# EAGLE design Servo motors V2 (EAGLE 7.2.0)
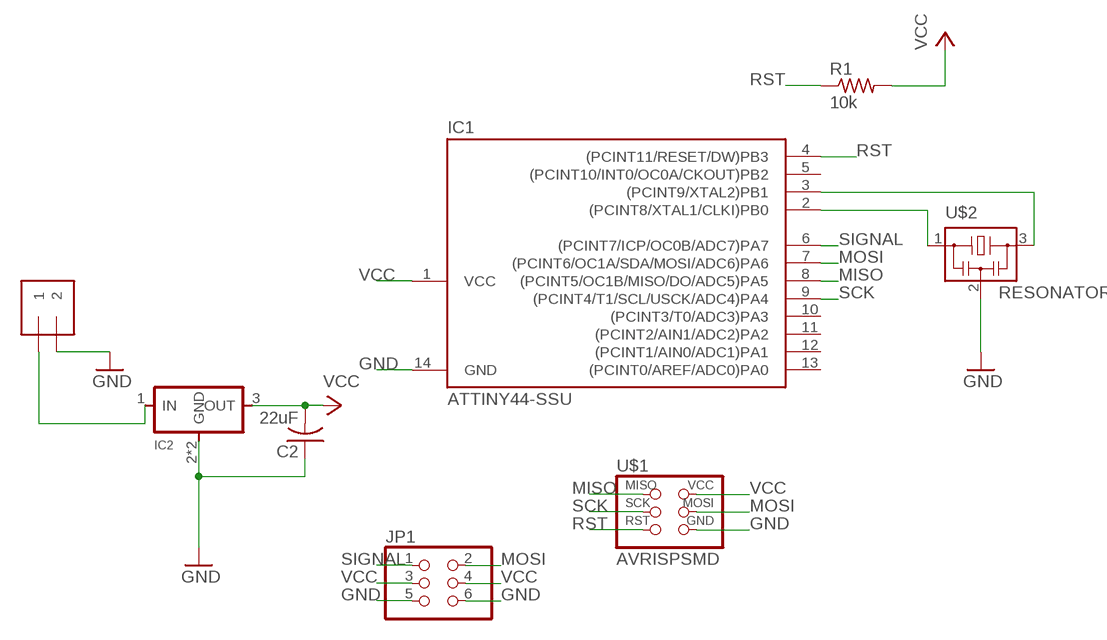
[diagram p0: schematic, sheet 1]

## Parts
C2  22uF  C-USC1206  [C1206]
IC1  ATTINY44-SSU  [SOIC14]
IC2  REGULATORSOT223  [SOT223]
J1  1X2-3.5MM  [3.5MMTERM]
JP1  PINHD-2X3-SMD  [2X03SMD]
R1  10k  RESISTOR1206  [1206]
U$1  AVRISPSMD  [2X03SMD]
U$2  RESONATOR  [EFOBM]

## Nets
GND: C2.1 IC1.14(GND) IC2.2(GND) IC2.4(GND) J1.2 JP1.5 JP1.6 U$1.6(GND) U$2.2
MISO: IC1.8((PCINT5/OC1B/MISO/DO/ADC5)PA5) U$1.1(MISO)
MOSI: IC1.7((PCINT6/OC1A/SDA/MOSI/ADC6)PA6) JP1.2 U$1.4(MOSI)
N$1: IC1.3((PCINT9/XTAL2)PB1) U$2.3
N$2: IC1.2((PCINT8/XTAL1/CLKI)PB0) U$2.1
N$3: IC2.1(IN) J1.1
RST: IC1.4((PCINT11/RESET/DW)PB3) R1.1 U$1.5(RST)
SCK: IC1.9((PCINT4/T1/SCL/USCK/ADC4)PA4) U$1.3(SCK)
SIGNAL: IC1.6((PCINT7/ICP/OC0B/ADC7)PA7) JP1.1
VCC: C2.2 IC1.1(VCC) IC2.3(OUT) JP1.3 JP1.4 R1.2 U$1.2(VCC)
Unconnected: IC1.5((PCINT10/INT0/OC0A/CKOUT)PB2) IC1.10((PCINT3/T0/ADC3)PA3) IC1.11((PCINT2/AIN1/ADC2)PA2) IC1.12((PCINT1/AIN0/ADC1)PA1) IC1.13((PCINT0/AREF/ADC0)PA0)

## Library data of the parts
C2 = 01_adafruit:C-US: CAPACITOR, American symbol
IC1 = 01_FAB_Hello:ATTINY44
IC2 = 01_fab:REGULATOR
J1 = 01_adafruit:1X2: 3.5mm Terminal block
JP1 = 01_FAB_Hello:PINHD-2X3-SMD: PIN HEADER
R1 = 01_FAB_Hello:RESISTOR
U$1 = 01_FAB_Hello:AVRISP
U$2 = 01_fab:RESONATOR

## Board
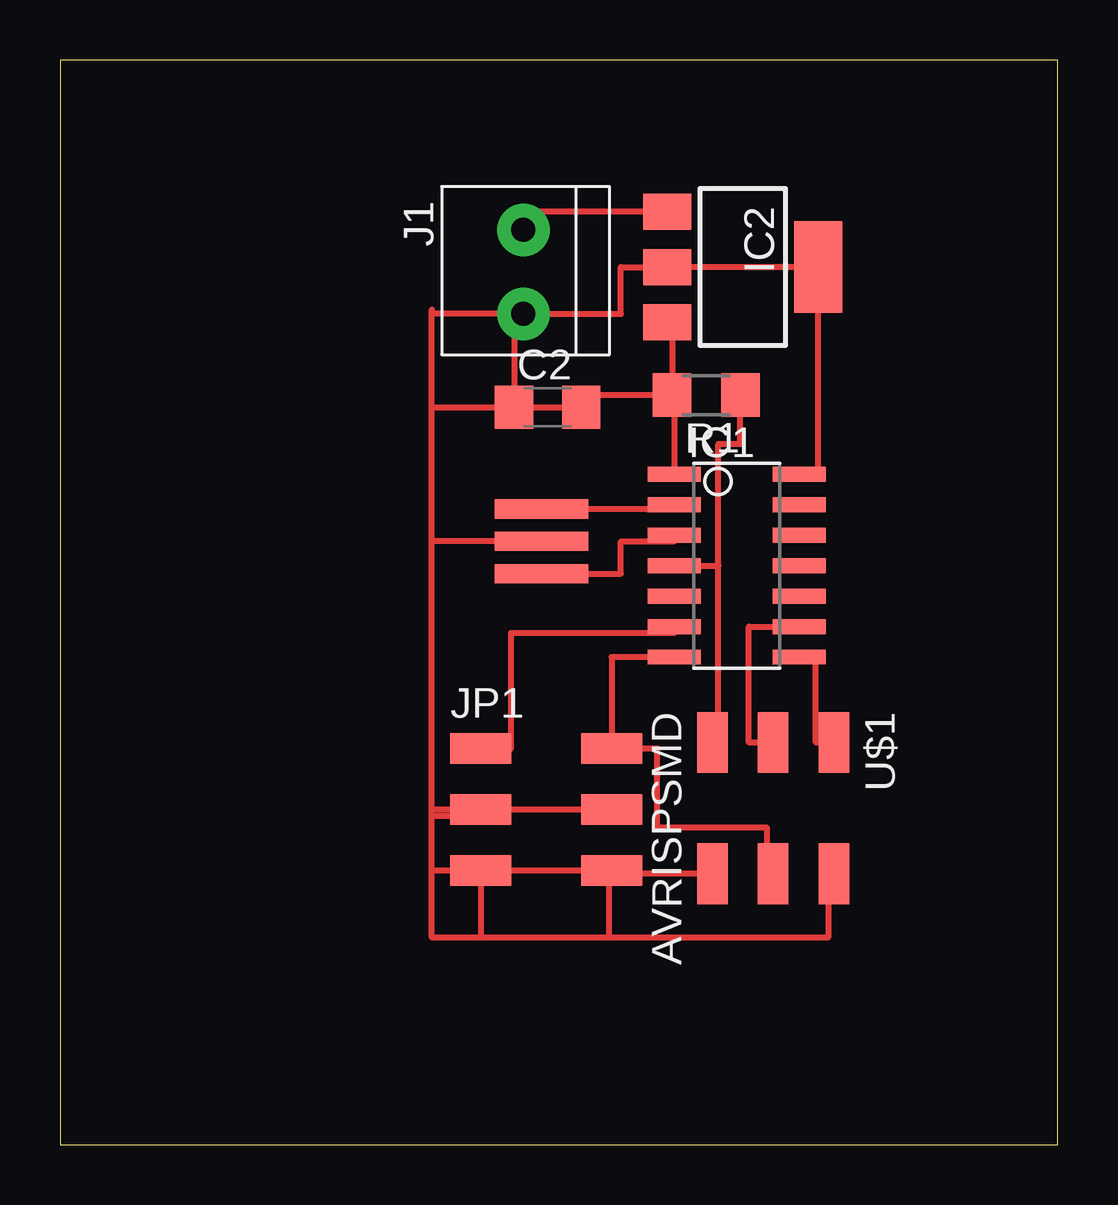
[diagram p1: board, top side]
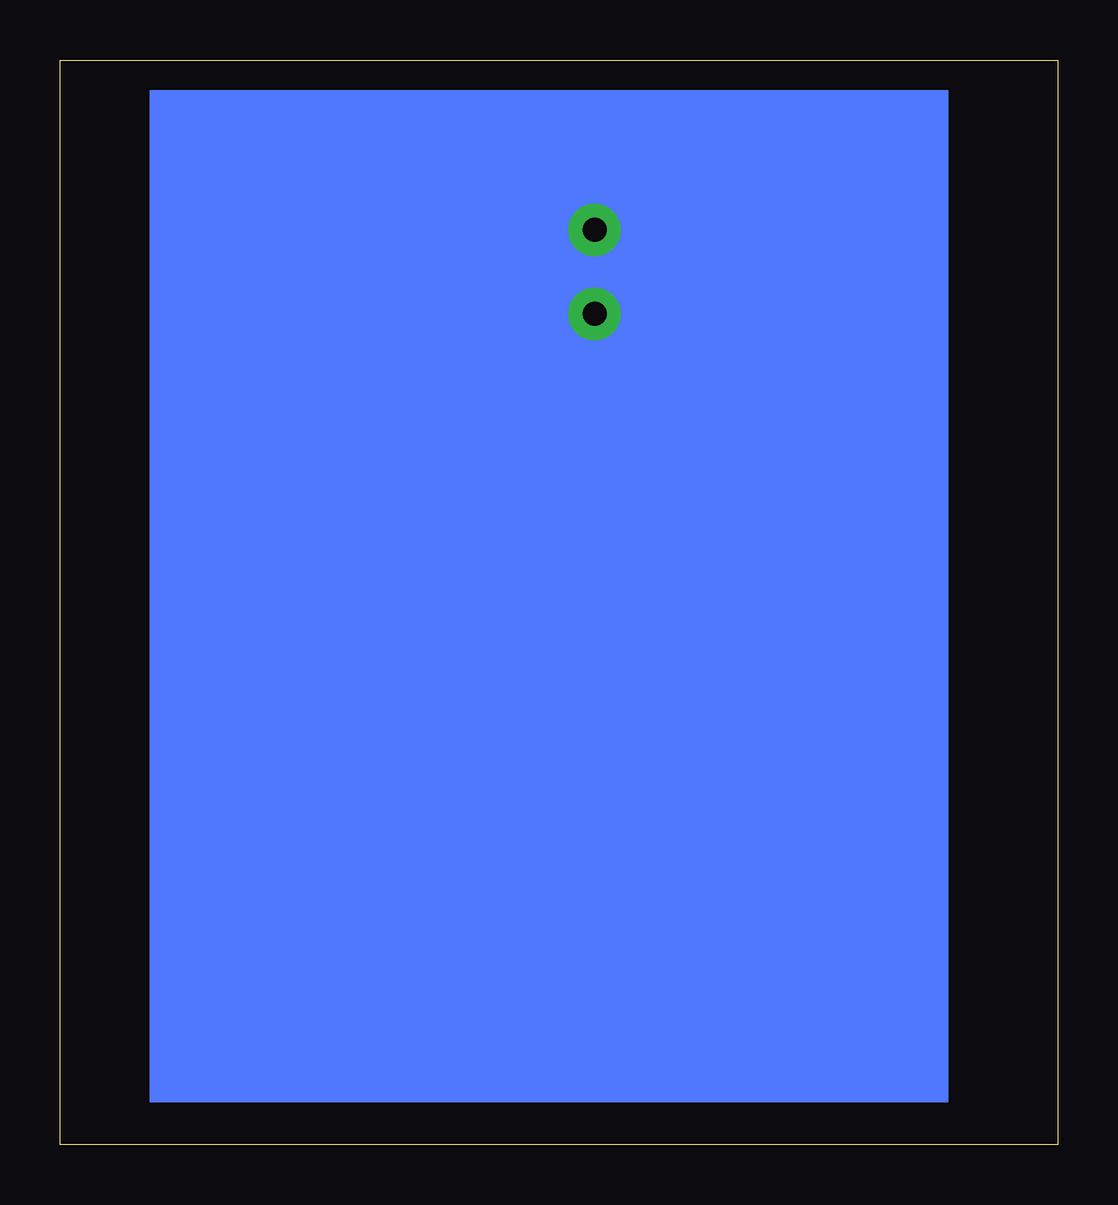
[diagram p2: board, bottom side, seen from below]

Size 41.58 x 45.2 mm. Coordinates in mm from the lower left corner, seen from the top.
Outline: 0,0 41.58,0 41.58,45.2 0,45.2 0,0
Copper layers (1*16): Top 0.035mm / dielectric 1.5mm / Bottom 0.035mm
Design rules "fabmodule": minimum track width 10mil, minimum drill 0.4mm, track to track 0.42mm, track to pad 0.42mm, pad to pad 0.42mm, via to via 0.42mm, smd to smd 0.42mm, copper to edge 40mil, drill to drill 0.8mm, minimum pad ring 10mil, minimum via ring 8mil, stop-mask expansion 4mil, vias tented up to drill 0mil, thermal gap 10mil

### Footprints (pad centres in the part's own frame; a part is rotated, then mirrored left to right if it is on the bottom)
C1206 = smd 1.6 x 1.8: 1 -1.4,0; 2 1.4,0
SOIC14 = smd 0.61 x 2.21: 1 -3.81,-2.603; 2 -2.54,-2.603; 3 -1.27,-2.603; 4 0,-2.603; 5 1.27,-2.603; 6 2.54,-2.603; 7 3.81,-2.603; 8 3.81,2.603; 9 2.54,2.603; 10 1.27,2.603; 11 0,2.603; 12 -1.27,2.603; 13 -2.54,2.603; 14 -3.81,2.603
SOT223 = smd 1.5 x 2: 1 -2.3,-3.15; 2 0,-3.15; 3 2.3,-3.15 | smd 3.8 x 2: 4 0,3.15
3.5MMTERM = drill 1 pad 2.184: 1 1.8,0; 2 -1.7,0
2X03SMD = smd 2.54 x 1.27: 1 -2.54,2.54; 2 2.92,2.54; 3 -2.54,0; 4 2.92,0; 5 -2.54,-2.54; 6 2.92,-2.54
1206 = smd 1.6 x 1.803: 1 -1.422,0; 2 1.422,0
EFOBM = smd 0.8 x 3.9: 1 -1.35,0; 2 0,0; 3 1.35,0

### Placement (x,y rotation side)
C2  20.32,30.73 0 top
IC1  28.19,24.13 270 top
IC2  28.45,36.58 270 top
J1  19.3,36.32 90 top
JP1  20.07,13.97 0 top
R1  26.92,31.24 180 top
U$1  29.72,14.22 270 top
U$2  20.07,25.15 270 top

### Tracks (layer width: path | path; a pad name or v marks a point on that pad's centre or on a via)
GND
  Top 0.254: IC1.14 31.6,27.94 IC2.4 IC2.2 23.37,36.58 23.37,34.62 J1.2 | U$2.2 15.49,25.15 | 15.49,25.15 15.49,34.62 | JP1.5 17.53,8.64 | JP1.6 22.86,11.43 22.86,8.64 | JP1.6 JP1.5 | U$1.6 22.99,11.3 JP1.6 | JP1.5 15.49,11.43 15.49,25.15 | J1.2 15.49,34.62 | 15.49,34.62 15.49,34.8 | J1.2 18.92,34.62 C2.1
MISO
  Top 0.254: U$1.1 31.5,16.76 31.5,20.32 | 31.5,20.32 31.75,20.32 | 31.5,20.32 IC1.8
MOSI
  Top 0.254: U$1.4 29.46,11.3 29.46,13.21 24.89,13.21 24.89,16.51 JP1.2 22.99,20.32 IC1.7
N$1
  Top 0.254: U$2.3 23.37,23.8 23.37,25.15 25.59,25.15 IC1.3
N$2
  Top 0.254: U$2.1 25.59,26.5 IC1.2
N$3
  Top 0.254: IC2.1 19.3,38.88 J1.1
RST
  Top 0.254: U$1.5 27.43,16.76 27.43,24.13 | IC1.4 27.43,24.13 | 27.43,24.13 27.43,29.21 28.35,29.21 R1.1
SCK
  Top 0.254: U$1.3 28.7,16.76 28.7,21.59 IC1.9
SIGNAL
  Top 0.254: JP1.1 18.8,16.51 18.8,21.34 25.59,21.34 IC1.6
VCC
  Top 0.254: U$1.2 32,11.3 32,8.64 15.49,8.64 15.49,13.72 17.53,13.72 JP1.3 | JP1.3 15.49,13.97 15.49,30.73 19.05,30.73 | 19.05,30.99 19.05,30.73 | 19.05,30.73 C2.2 21.72,31.24 R1.2 | IC2.3 25.5,34.28 R1.2 | R1.2 25.59,31.24 IC1.1 | JP1.4 JP1.3
(copper drawn outside any net)
  shapes: Bottom area x1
